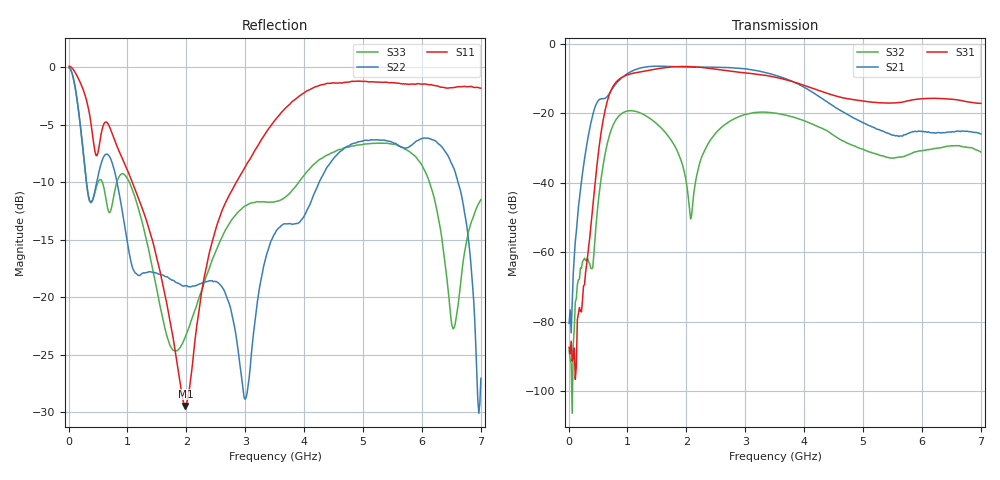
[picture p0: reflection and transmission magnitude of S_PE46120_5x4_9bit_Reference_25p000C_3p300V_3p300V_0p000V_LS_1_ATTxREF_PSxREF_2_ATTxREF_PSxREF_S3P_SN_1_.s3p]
! Device ID: PE46120_5x4_9bit_Reference
! Device ID: PE46120_5x4_9bit_Reference
! File Path: z:\PE46120_5x4_9bit_Reference\MPAC_Yi\new_12port\25p000C\3p300\LS_1_ATTxREF_PSxREF_2_ATTxREF_PSxREF\PE46120_5x4_9bit_Reference_25p000C_3p300V_3p300V_0p000V_LS_1_ATTxREF_PSxREF_2_ATTxREF_PSxREF_S3P_SN_1_.s3p
! Serial: 1
! Lot:
! Temp: 25.000C
! VDD: 3.300
! VSS: 0.000
! Control_Hi: 3.300
! Control_Lo: 0.000
! Logic State: LS_1_ATTxREF_PSxREF_2_ATTxREF_PSxREF
! Port 1: RFin
! Port 2: RFout1
! Port 3: RFout2
! ThroughPath:1-2
! IDD: -0.0005457338
! ISS: 0
! Comment:
#  Hz  S  RI  R  50
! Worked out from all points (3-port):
!   401 points, 10 MHz to 7 GHz, reference 50 ohm
!   strongest paths, dB at 10 MHz, 1.758 GHz, 3.505 GHz, 5.253 GHz, 7 GHz:
!     S31: -87.4, -6.7, -9.6, -17.0, -17.2
!     S21: -80.5, -6.6, -9.1, -24.7, -26.0
!     S32: -88.3, -28.2, -20.0, -31.9, -31.2
!   lowest |S11| = -29.5 dB at 1.985 GHz (marker M1), VSWR 1.07, Z = 53 + j1.81 ohm
!   |S11| at or under -10 dB: 1.082 GHz to 2.849 GHz (1.767 GHz wide, 89.9 % of centre)
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1e7  1.002 -0.1146  1.04e-06 -9.31e-05  -7.71e-05 -2.92e-05
     8.38e-05 -4.25e-05  0.9887 -0.0954  7.76e-07 7.33e-06
     -3.68e-05 -2.13e-05  -3.04e-05 2.33e-05  0.9879 -0.0961
2.37175e8  -0.4737 -0.6596  -0.0126 -0.00508  0.000104 0.000215
           -0.0126 -0.00531  -0.2914 -0.3539  -0.000346 0.000746
           7.56e-05 0.000189  -0.000387 0.000611  -0.2932 -0.3492
4.81825e8  -0.401 -0.0925  -0.0421 0.1333  0.0171 0.00274
           -0.0423 0.135  0.1901 0.2552  -0.0022 0.00252
           0.0174 0.00266  -0.00226 0.00254  0.206 0.2269
9.5365e8  -0.2779 0.2573  0.3363 -0.0713  -0.0886 0.3284
          0.3405 -0.0727  -0.0504 -0.1957  -0.0486 0.0913
          -0.0886 0.332  -0.0487 0.0923  0.1019 -0.3243
1.984675e9  0.029 0.017  -0.3681 0.2678  -0.2847 -0.3668
            -0.3724 0.2716  -0.0908 0.0658  0.00194 0.0115
            -0.2892 -0.3701  0.00203 0.0118  -0.0673 0.00203
2.806e9  -0.0786 -0.2915  0.4335 0.0934  -0.0968 0.38
         0.4396 0.0934  0.0717 -0.0277  0.0128 0.0809
         -0.0967 0.3846  0.0133 0.0815  0.0666 0.2119
3.505e9  -0.4372 -0.3929  -0.0901 -0.336  0.3225 0.0493
         -0.0918 -0.3403  0.0628 0.1785  0.0104 -0.0987
         0.3264 0.0492  0.0107 -0.0998  0.1853 -0.182
4.605925e9  -0.851 0.0564  -0.00846 0.1085  -0.0723 -0.1527
            -0.00833 0.1103  -0.3995 0.1538  0.0293 0.0303
            -0.0734 -0.1541  0.0294 0.03  -0.2751 0.3413
6.248575e9  -0.3732 0.7393  0.0403 -0.0317  -0.0175 0.1609
            0.0406 -0.0323  0.4633 -0.0948  -0.0304 -0.00706
            -0.017 0.1626  -0.0305 -0.00717  0.2057 -0.1268
7e9  -0.1135 0.8012  -0.0295 -0.0401  0.1241 0.0563
     -0.0296 -0.0408  -0.0372 0.0243  0.026 0.00931
     0.1262 0.0564  0.0262 0.00866  0.1473 0.2208
